TYPE E_PMLUnitMode : (
	ePMLUnitMode_UNDEFINED		:=  0,
	ePMLUnitMode_AUTOMATIC		:=  1,
	ePMLUnitMode_MAINTENANCE 	:=  2,
	ePMLUnitMode_MANUAL 		:=  3,
	ePMLUnitMode_SEMIAUTOMATIC	:=  4,
	ePMLUnitMode_DRYRUN			:=  5,
	ePMLUnitMode_USERMODE1		:=  6,
	ePMLUnitMode_USERMODE2		:=  7,
	ePMLUnitMode_IDLE 			:=  8,
	ePMLUnitMode_ESTOP 			:=  9
);
END_TYPE
